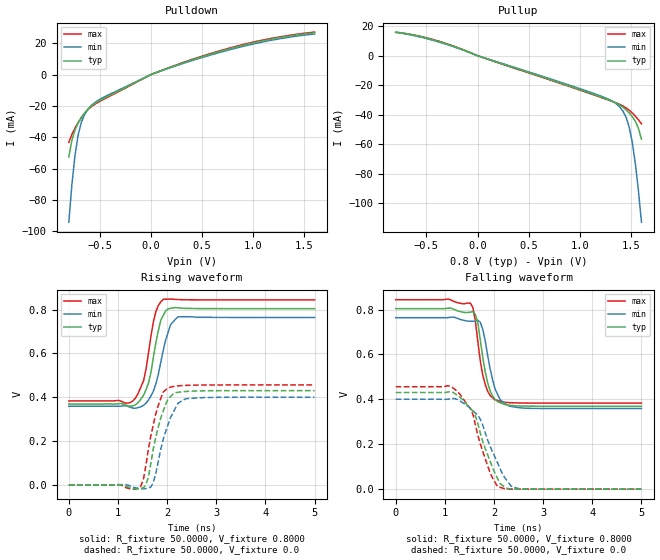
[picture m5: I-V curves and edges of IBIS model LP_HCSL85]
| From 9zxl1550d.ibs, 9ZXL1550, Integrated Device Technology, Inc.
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|   Model LP_HCSL85   (lphcsl_0v8_fast 85 ohm)
[Model]  LP_HCSL85
Model_type Output
Polarity   Non-Inverting
Vmeas =  0.4000V
Cref =   2.0000pF
Rref =   0.0
Vref =   0.4000V
C_comp   1.1000pF   1.0000pF   1.2000pF
[Temperature Range]   27.0000   70.0000   0.0
[Voltage Range]   0.8000V   0.7600V   0.8400V
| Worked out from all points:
|   slope of the pulldown table from 0 to 0.12 V, typ, clamps not added: 39.7 ohm
|   slope of the pullup table from 0 to 0.12 V, typ, clamps not added: 43 ohm
|   rising waveform, R_fixture 50.0000, V_fixture 0.8000: 20-80 % time 228ps typ, 263ps min, 209ps max; typ from 0.37 V to 0.804 V
|   rising waveform, R_fixture 50.0000, V_fixture 0.0: 20-80 % time 274ps typ, 304ps min, 255ps max; typ from 0 V to 0.43 V
|   falling waveform, R_fixture 50.0000, V_fixture 0.8000: 20-80 % time 209ps typ, 235ps min, 192ps max; typ from 0.804 V to 0.37 V
|   falling waveform, R_fixture 50.0000, V_fixture 0.0: 20-80 % time 412ps typ, 452ps min, 393ps max; typ from 0.43 V to 0 V
[Pulldown]
|Voltage   I(typ)   I(min)   I(max)
-800mV    -52.6mA    -94.18mA   -43.24mA
-770mV    -41.91mA   -70.21mA   -38.14mA
-740mV    -35.37mA   -51.69mA   -34.18mA
-710mV    -30.97mA   -38.94mA   -30.73mA
-680mV    -27.6mA    -30.95mA   -27.68mA
-650mV    -24.82mA   -26mA      -25.03mA
-620mV    -22.5mA    -22.72mA   -22.8mA
-560mV    -19.01mA   -18.52mA   -19.5mA
10mV      253uA      240uA      261uA
430mV     9.97mA     9.528mA    10.28mA
1.03V     20.72mA    19.97mA    21.2mA
1.6V      26.71mA    25.98mA    27.17mA
[Pullup]
|Voltage   I(typ)   I(min)   I(max)
-800mV    15.86mA    15.71mA    15.69mA
-560mV    12.86mA    12.51mA    12.97mA
-320mV    8.215mA    7.894mA    8.391mA
1.12V     -26.02mA   -25.38mA   -26.33mA
1.36V     -32.44mA   -33.07mA   -32.3mA
1.42V     -35.09mA   -37.77mA   -34.22mA
1.45V     -36.85mA   -41.89mA   -35.49mA
1.48V     -38.92mA   -48.47mA   -37.05mA
1.51V     -41.42mA   -58.66mA   -38.91mA
1.54V     -44.6mA    -73.03mA   -41.07mA
1.57V     -49.22mA   -91.31mA   -43.51mA
1.6V      -56.61mA   -112.9mA   -46.27mA
[Ramp]
| variable   typ   min   max
dV/dt_r  0.2583/0.2739n   0.2404/0.3037n   0.2739/0.2552n
dV/dt_f  0.2593/0.2088n   0.2352/0.2353n   0.2758/0.1918n
R_load = 50.0000
[Rising Waveform]
R_fixture= 50.0000
V_fixture= 0.8000
V_fixture_min= 0.7600
V_fixture_max= 0.8400
|time   V(typ)   V(min)   V(max)
0s        369.5mV    359.4mV    383.5mV
1.31ns    361.8mV    350.8mV    384.8mV
1.52ns    409.6mV    363.4mV    475.2mV
1.62ns    464.6mV    387.9mV    601.7mV
1.77ns    647.6mV    461.1mV    790mV
1.87ns    750.5mV    559.4mV    834.8mV
1.92ns    773mV      613.6mV    846.8mV
2.07ns    805.7mV    730.9mV    847.9mV
2.22ns    808mV      767mV      845.6mV
5ns       804.2mV    764.1mV    844.2mV
[Rising Waveform]
R_fixture= 50.0000
V_fixture= 0.0
V_fixture_min= 0.0
V_fixture_max= 0.0
|time   V(typ)   V(min)   V(max)
0s        423.2nV    0V         514.2nV
1.46ns    -16.05mV   -16.23mV   -6.751mV
1.52ns    -11.89mV   -16.75mV   28.07mV
1.57ns    2.593mV    -15.93mV   93.03mV
1.72ns    167mV      12.7mV     276.8mV
1.92ns    336.7mV    207.9mV    424.4mV
2.02ns    392.8mV    277mV      442.4mV
2.22ns    422.7mV    372.5mV    452.2mV
2.42ns    427.2mV    394.4mV    454.8mV
5ns       430.5mV    400.6mV    456.5mV
[Falling Waveform]
R_fixture= 50.0000
V_fixture= 0.8000
V_fixture_min= 0.7600
V_fixture_max= 0.8400
|time   V(typ)   V(min)   V(max)
0s        804.2mV    764.1mV    844.2mV
1.52ns    789.1mV    748mV      828.5mV
1.57ns    790.6mV    748mV      810.1mV
1.62ns    778.9mV    749.6mV    750.4mV
1.72ns    666.5mV    744.1mV    573.4mV
1.87ns    474.7mV    597.1mV    436.6mV
2.02ns    400.8mV    447.4mV    398.1mV
2.17ns    381.3mV    389.4mV    388.9mV
2.53ns    370.4mV    362.2mV    383.9mV
5ns       369.5mV    359.4mV    383.5mV
[Falling Waveform]
R_fixture= 50.0000
V_fixture= 0.0
V_fixture_min= 0.0
V_fixture_max= 0.0
|time   V(typ)   V(min)   V(max)
0s        430.5mV    400.6mV    456.5mV
1.06ns    432.9mV    400.7mV    460.6mV
1.26ns    417.4mV    398.5mV    433.7mV
1.52ns    360.1mV    360.5mV    359.5mV
1.62ns    327.6mV    339.4mV    288.5mV
1.92ns    124.7mV    190.6mV    73.1mV
2.07ns    48.43mV    118.1mV    12.09mV
2.37ns    922uV      8.403mV    269.7uV
2.53ns    419.6uV    1.087mV    51.4uV
5ns       584.9nV    0V         596.8nV
